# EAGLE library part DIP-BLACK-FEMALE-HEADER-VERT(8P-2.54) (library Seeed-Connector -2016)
320030061
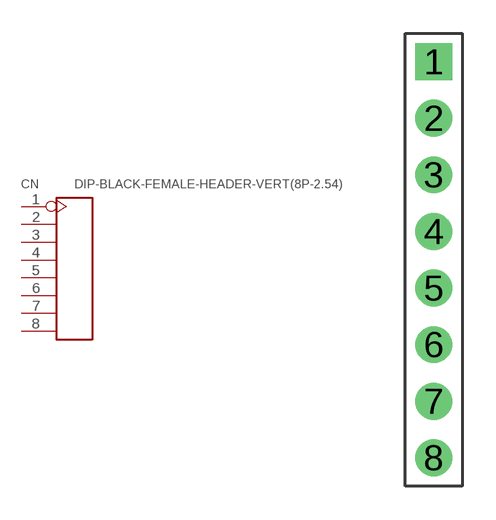
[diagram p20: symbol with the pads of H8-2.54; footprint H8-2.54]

Designator prefix CN

## DIP-BLACK-FEMALE-HEADER-VERT(8P-2.54) (MPN: F185-1108A1BSYC1; VALUE: 8p-2.54)  [H8-2.54]
1  1
2  2
3  3
4  4
5  5
6  6
7  7
8  8

## Footprint H8-2.54 (pad centres in mm)
drill 0.889 pad 1.651 square: 1 0,8.89
drill 0.889 pad 1.651: 2 0,6.35; 3 0,3.81; 4 0,1.27; 5 0,-1.27; 6 0,-3.81; 7 0,-6.35; 8 0,-8.89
